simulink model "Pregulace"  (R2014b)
settings: Solver=ode4  SolverMode=SingleTasking  StartTime=0.0  StopTime=30  FixedStep=0.001  RelTol=1e-3
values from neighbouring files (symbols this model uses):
  dS = [parS(2)*parS(3)^2, (2*parS(4)*parS(2)*parS(3)+parS(3)^2), parS(2)+2*parS(4)*parS(3), 1]    [tlumeniP.m]    (also in tlumeniPD.m)
  Kp = -8    [tlumeniP.m]    (also in SITOrizeniP.m = -4.5; SITOrizeniPD.m = -4; tlumeniPD.m = -6)
  parS = [-0.0628 0.17 0.22 0.0318]    [tlumeniP.m]    (also in tlumeniPD.m)
libraries: simulink x1

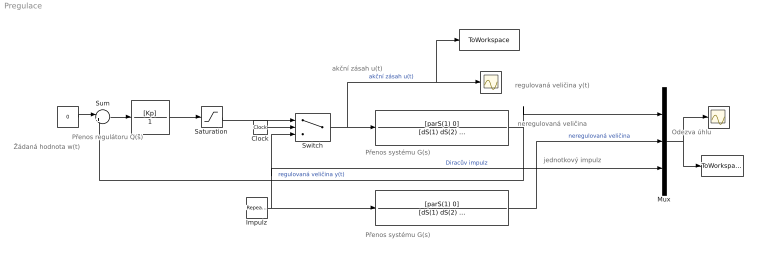
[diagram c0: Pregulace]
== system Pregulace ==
  note: Odezva úhlu
  note: neregulovaná veličina
  note: jednotkový impulz
  note: akční zásah u(t)
  note: Přenos systému G(s)
  note: Přenos systému G(s)
  note: Přenos regulátoru Q(s)
  note: Žádaná hodnota w(t)
  note: regulovaná veličina y(t)
  "  " : Constant  Value=0
  "    " : TransferFcn  Numerator=[Kp]  Denominator=1
  "     " : TransferFcn  Numerator=[parS(1) 0]  Denominator=[dS(1) dS(2) dS(3) dS(4)]
  "         " : Scope
  "                         " : TransferFcn  Numerator=[parS(1) 0]  Denominator=[dS(1) dS(2) dS(3) dS(4)]
  "                                 " : ToWorkspace  VariableName=dataPreg  SaveFormat=Timeseries  SampleTime=-1
  "                                           " : Scope
  "                                                                                  " : ToWorkspace  VariableName=akcniZasahPreg  SaveFormat=Timeseries  SampleTime=-1
  Clock : Clock
  Impulz : simulink/Sources/Repeating Sequence  rep_seq_t=[0 2.99 3 3.99 4 40]  rep_seq_y="[0  0     1   1    0      0]"
  Mux : Mux  Inputs=3
  Saturation : Saturate  UpperLimit=1  LowerLimit=-1
  Sum : Sum  Inputs=|+-
  Switch : Switch  Threshold=8
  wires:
  "  "/1 -> Sum/1
  "     "/1 -> Sum/2, Mux/1  "regulovaná veličina y(t)"
  "    "/1 -> Saturation/1
  Sum/1 -> "    "/1
  Impulz/1 -> "                         "/1, Mux/3, Switch/3  "Diracův impulz"
  Mux/1 -> "                                 "/1, "         "/1
  Switch/1 -> "                                           "/1, "                                                                                  "/1, "     "/1  "akční zásah u(t)"
  Saturation/1 -> Switch/1
  Clock/1 -> Switch/2
  "                         "/1 -> Mux/2  "neregulovaná veličina"
